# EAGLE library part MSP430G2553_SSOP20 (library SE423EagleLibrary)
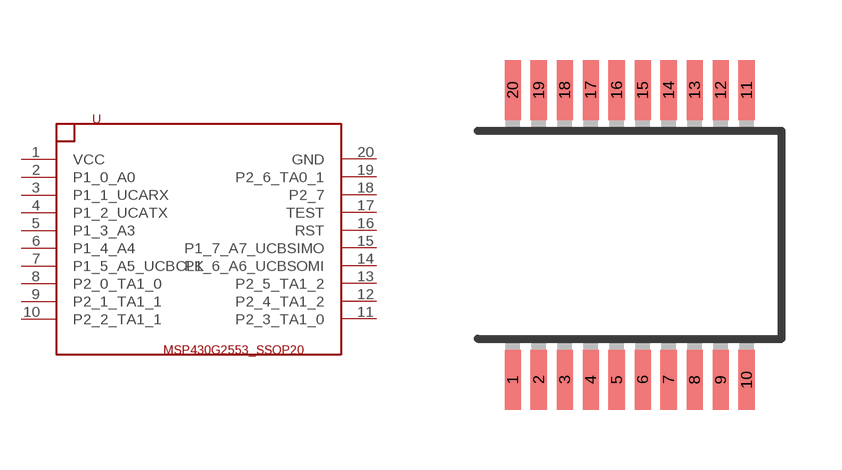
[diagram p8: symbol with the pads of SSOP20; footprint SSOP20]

Designator prefix U

## MSP430G2553_SSOP20  [SSOP20]
1  VCC
2  P1_0_A0
3  P1_1_UCARX
4  P1_2_UCATX
5  P1_3_A3
6  P1_4_A4
7  P1_5_A5_UCBCLK
8  P2_0_TA1_0
9  P2_1_TA1_1
10  P2_2_TA1_1
11  P2_3_TA1_0
12  P2_4_TA1_2
13  P2_5_TA1_2
14  P1_6_A6_UCBSOMI
15  P1_7_A7_UCBSIMO
16  RST
17  TEST
18  P2_7
19  P2_6_TA0_1
20  GND

## Footprint SSOP20 (pad centres in mm)
Shrink Small Outline Package package type SS
smd 0.4 x 1.5: 1 -2.925,-3.625; 2 -2.275,-3.625; 3 -1.625,-3.625; 4 -0.975,-3.625; 5 -0.325,-3.625; 6 0.325,-3.625; 7 0.975,-3.625; 8 1.625,-3.625; 9 2.275,-3.625; 10 2.925,-3.625; 11 2.925,3.625; 12 2.275,3.625; 13 1.625,3.625; 14 0.975,3.625; 15 0.325,3.625; 16 -0.325,3.625; 17 -0.975,3.625; 18 -1.625,3.625; 19 -2.275,3.625; 20 -2.925,3.625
